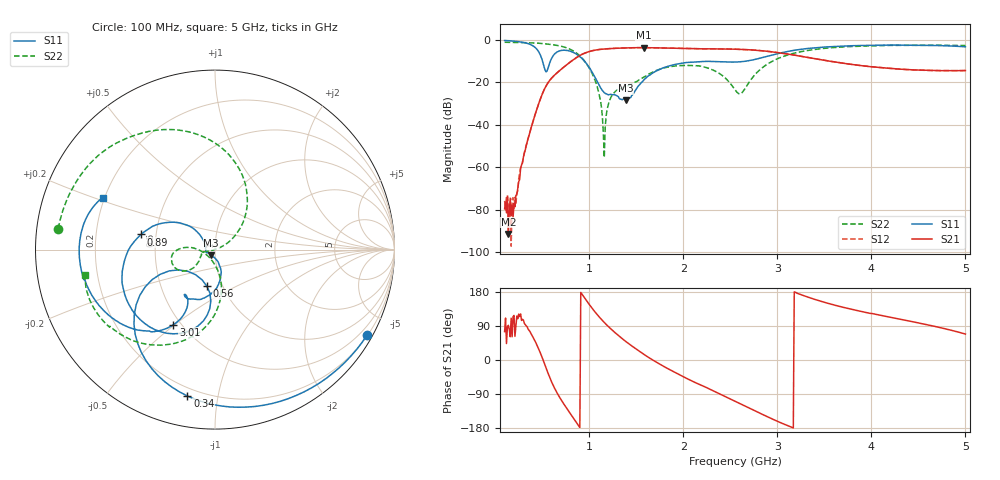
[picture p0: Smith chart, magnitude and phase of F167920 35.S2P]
!  2-Port S-parameters saved by WinCal
! VAR MeasName=S-Parameters (CALIBRATED_DATA) read from VNA (N5242A)
! VAR MeasDate=2016-11-22 9:57:08
! VAR NAME=F167920 35
! VAR FILENAME=F167920 35.S2P
! VAR DATE=2016-11-22 9:57:08
! VAR PHYS_PORTS=1,2
# Hz S DB R 50
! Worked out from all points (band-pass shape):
!   491 points, 100 MHz to 5 GHz, reference 50 ohm
!   highest |S21| = -3.64 dB at 1.58 GHz (marker M1); lowest = -91.5 dB at 140 MHz (marker M2)
!   |S21| within 3 dB of the highest: 931.1 MHz to 3.109 GHz (2.178 GHz wide, 108 % of centre)
!   lowest |S11| = -28.5 dB at 1.39 GHz (marker M3), VSWR 1.08, Z = 47.9 - j3 ohm
!   |S11| at or under -10 dB: 503.3 MHz to 586.8 MHz (83.48 MHz wide, 15.3 % of centre); 948.5 MHz to 2.669 GHz (1.721 GHz wide, 95.1 % of centre)
!   |S22| runs from -55.4 to -1.1 dB; largest |S21 - S12| = 0.0015
!   S11 on the Smith chart (normalised r, x): 100 MHz: 0.22, -3.82; 340 MHz: 0.16, -0.82; 560 MHz: 0.84, -0.36; 890 MHz: 0.41, +0.08; 3.01 GHz: 0.46, -0.49; 5 GHz: 0.19, +0.21
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1e8  -0.25 -29.3  -79.59 74.9  -75.90 84.6  -1.10 172.4
1.4e8  -0.37 -40.7  -91.46 91.6  -77.46 103.9  -1.12 169.3
2.2e8  -0.67 -63.8  -73.32 90.3  -77.52 107.4  -1.19 163.1
3.4e8  -1.62 -100.7  -48.17 87.5  -48.05 88.0  -1.32 153.1
4.5e8  -4.78 -141.2  -31.72 36.1  -31.67 36.2  -1.53 142.4
5.6e8  -13.59 -102.5  -20.32 -33.6  -20.32 -33.7  -1.97 129.9
6.8e8  -5.22 -123.2  -14.65 -96.4  -14.65 -96.4  -2.77 113.2
8.9e8  -7.53 168.4  -7.63 -174.5  -7.62 -174.5  -7.10 69.8
9.2e8  -8.60 159.5  -6.87 174.7  -6.86 174.7  -8.42 62.6
1.08e9  -19.20 136.4  -4.69 121.1  -4.68 121.1  -21.38 28.7
1.16e9  -24.92 161.9  -4.27 99.0  -4.26 99.0  -55.44 148.7
1.23e9  -25.66 -170.4  -4.07 82.0  -4.07 82.0  -27.11 -167.2
1.39e9  -28.54 -123.4  -3.77 48.8  -3.77 48.8  -21.79 -161.1
1.58e9  -18.93 -73.6  -3.64 15.1  -3.64 15.1  -17.59 -141.0
1.74e9  -14.04 -84.9  -3.77 -9.5  -3.77 -9.5  -13.98 -143.9
2.21e9  -10.17 -117.7  -4.22 -68.5  -4.21 -68.5  -12.60 -174.9
2.55e9  -10.43 -122.6  -4.35 -108.5  -4.35 -108.5  -23.44 -166.3
2.62e9  -10.25 -120.4  -4.46 -116.8  -4.45 -116.8  -25.07 -119.0
3.01e9  -6.40 -119.0  -6.01 -162.7  -6.00 -162.8  -8.73 -90.6
3.37e9  -3.82 -137.6  -8.62 162.2  -8.60 162.1  -4.66 -115.6
4.19e9  -2.43 -174.6  -13.40 113.3  -13.41 113.1  -2.58 -149.6
5e9  -3.24 155.2  -14.43 68.4  -14.44 68.2  -2.65 -168.8
